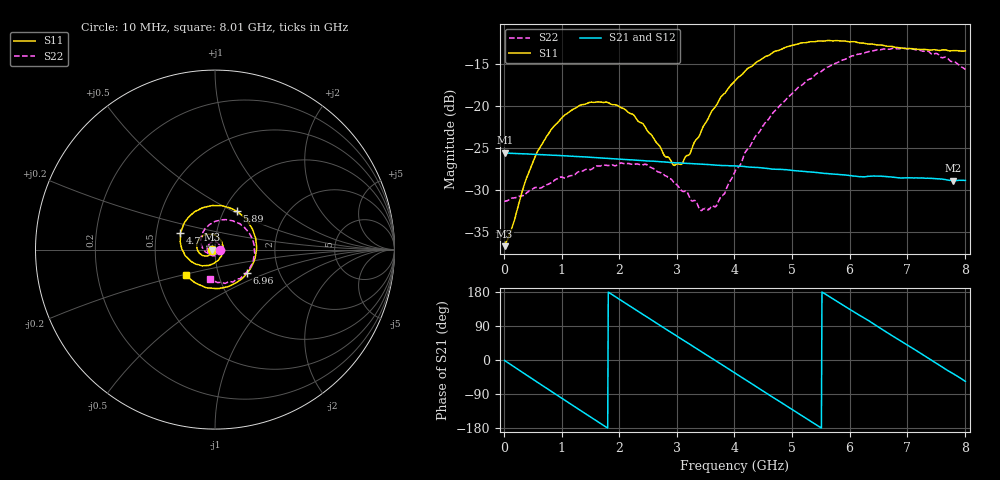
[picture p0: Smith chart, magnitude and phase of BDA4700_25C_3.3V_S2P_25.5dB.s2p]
!Agilent Technologies,E5071B,MY42404982,A.09.10
!Date: Mon Oct 20 18:13:47 2025
!Data & Calibration Information:
!Freq	S11:SOLT2(ON)	S21:SOLT2(ON)	S12:SOLT2(ON)	S22:SOLT2(ON)
# Hz S RI R 50
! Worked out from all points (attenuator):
!   801 points, 10 MHz to 8.01 GHz, reference 50 ohm
!   highest |S21| = -25.57 dB at 20 MHz (marker M1); lowest = -28.9 dB at 7.8 GHz (marker M2)
!   lowest |S11| = -36.7 dB at 10 MHz (marker M3), VSWR 1.03, Z = 48.6 - j0.12 ohm
!   |S11| at or under -10 dB: start of sweep to end of sweep
!   |S22| runs from -32.5 to -13.0 dB; largest |S21 - S12| = 0.0006
!   S11 on the Smith chart (normalised r, x): 10 MHz: 0.97, -0.00; 4.7 GHz: 0.67, +0.13; 5.89 GHz: 1.15, +0.52; 6.96 GHz: 1.38, -0.37; 8.01 GHz: 0.70, -0.20
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1e7  -0.0145 -0.00123  0.0527 -0.00113  0.0527 -0.00115  0.0271 -0.000811
2e7  -0.0149 -0.00198  0.0527 -0.00201  0.0526 -0.00212  0.027 -0.00108
5.9e8  -0.0414 -0.0352  0.026 -0.0444  0.026 -0.0444  0.0139 -0.0295
1e9  -0.0814 -0.0247  -0.00929 -0.0498  -0.00926 -0.0498  -0.0146 -0.0348
1.35e9  -0.1017 0.0107  -0.0355 -0.0351  -0.0355 -0.0351  -0.0365 -0.0183
2.07e9  -0.0465 0.0852  -0.0432 0.0214  -0.0432 0.0214  -0.0309 0.0334
2.68e9  0.0351 0.0473  -0.00335 0.0466  -0.00346 0.0465  0.0129 0.0383
2.94e9  0.0442 0.00504  0.0165 0.0429  0.0165 0.0429  0.0254 0.0246
3.08e9  0.0405 -0.0195  0.0261 0.0377  0.0257 0.0378  0.0283 0.0135
3.41e9  0.00385 -0.0687  0.0414 0.0181  0.0414 0.0181  0.0212 -0.011
3.55e9  -0.0211 -0.0826  0.0441 0.00783  0.0442 0.00774  0.0131 -0.0202
3.7e9  -0.053 -0.0886  0.0443 -0.0034  0.0444 -0.00352  0.00027 -0.026
4.01e9  -0.1219 -0.0724  0.0363 -0.0249  0.0363 -0.0248  -0.0312 -0.0261
4.7e9  -0.1927 0.0906  -0.00837 -0.0412  -0.00818 -0.0413  -0.0795 0.0496
5.35e9  -0.059 0.236  -0.0389 -0.0109  -0.0388 -0.0112  -0.0161 0.1471
5.89e9  0.122 0.2129  -0.0316 0.0227  -0.0316 0.0226  0.1044 0.1582
6.28e9  0.2109 0.1086  -0.0121 0.0359  -0.0116 0.036  0.1847 0.0995
6.68e9  0.2254 -0.037  0.0132 0.0355  0.0132 0.0355  0.2191 0.000198
6.96e9  0.1797 -0.1291  0.0269 0.0258  0.027 0.0256  0.2093 -0.0749
7.41e9  0.0371 -0.2138  0.0371 0.000397  0.0372 0.000324  0.1267 -0.1637
7.8e9  -0.1043 -0.1884  0.0289 -0.0213  0.0289 -0.0213  0.02 -0.1834
8.01e9  -0.1623 -0.1402  0.02 -0.03  0.0202 -0.0299  -0.0301 -0.1632
